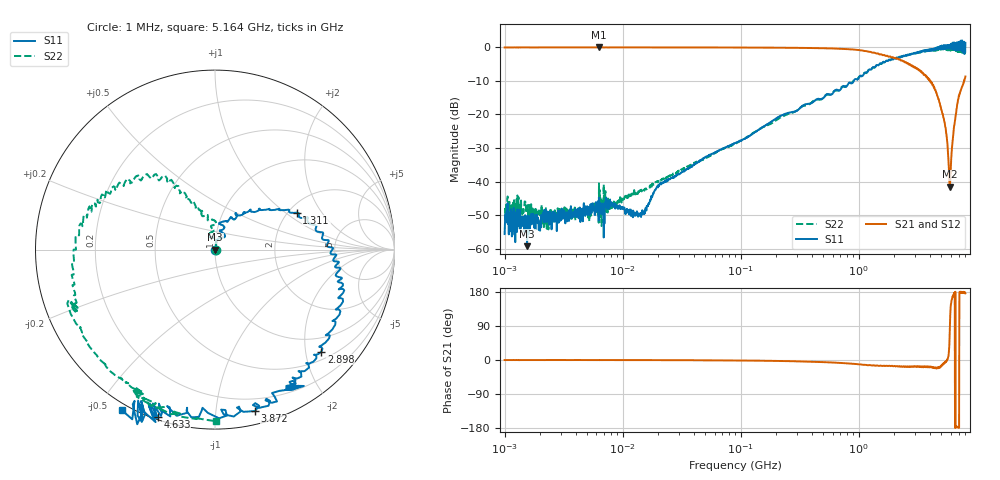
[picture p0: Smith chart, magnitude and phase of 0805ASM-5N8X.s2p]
!s-Parameter Generated by FASTRON Sdn. Bhd.
!FASTRON P/N : 0805ASM-5N8X
!Keysight Technologies: E5071C_MY46733604_B.14.02
!Date: Fri Jun 19 14:46:36 2026
!Version  :Rev00  Fri Jun 19 14:46:36 2026
!Data & Calibration Information:
!Freq  S11:SOLT2(ON)  S21:SOLT2(ON)  S12:SOLT2(ON)  S22:SOLT2(ON)
!PortZ  Port1:50+j0  Port2:50+j0
!When reading reference impedance value at option line is always used.
! Remarks : This data is being provided solely for informational purposes.
# Hz S dB R 50
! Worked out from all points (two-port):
!   1601 points, 1 MHz to 8 GHz, reference 50 ohm
!   highest |S21| = 0.01 dB at 6.301 MHz (marker M1); lowest = -41.5 dB at 5.918 GHz (marker M2)
!   |S21| within 3 dB of the highest: start of sweep to 1.886 GHz; 1.906 GHz to 1.955 GHz (49.23 MHz wide, 2.55 % of centre)
!   lowest |S11| = -59.2 dB at 1.55 MHz (marker M3), VSWR 1.00, Z = 50.1 - j0.0232 ohm
!   |S11| at or under -10 dB: start of sweep to 906.8 MHz
!   |S22| runs from -54.2 to -0.3 dB; largest |S21 - S12| = 0.0097
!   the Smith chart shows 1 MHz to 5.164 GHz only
!   S11 on the Smith chart (normalised r, x): 1 MHz: 1.00, -0.00; 1.311 GHz: 2.22, +1.22; 2.898 GHz: 0.67, -2.33; 3.872 GHz: 0.10, -1.27; 4.633 GHz: 0.01, -0.71; 5.164 GHz: -0.02, -0.58
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1000000  -55.60 -33.4  -0.04 -0.1  -0.03 -0.1  -49.20 -2.8
1066008  -52.60 13.6  -0.04 -0.1  -0.04 -0.0  -44.60 11.4
1550103  -59.20 -12.2  -0.03 -0.1  -0.03 -0.1  -48.00 -22.0
2173433  -48.90 24.8  -0.03 -0.1  -0.03 -0.0  -50.60 34.3
4479405  -49.80 21.3  -0.04 -0.1  -0.04 -0.1  -49.80 31.3
6301378  -44.80 33.3  0.01 -0.4  -0.00 -0.1  -40.50 41.1
1.414737e7  -49.30 64.4  -0.03 -0.3  -0.05 -0.3  -42.70 47.6
2.00676e7  -41.20 61.6  -0.04 -0.3  -0.05 -0.3  -39.90 66.8
8.994653e7  -28.50 78.6  -0.06 -1.3  -0.07 -1.2  -28.70 80.8
4.006501e8  -16.50 80.8  -0.22 -4.6  -0.22 -4.6  -16.30 87.9
1.310879e9  -6.02 24.3  -1.59 -14.2  -1.59 -14.3  -6.03 125.0
1.7949e9  -3.76 1.1  -2.81 -15.4  -2.81 -15.7  -3.73 145.0
2.472225e9  -2.49 -21.1  -4.53 -17.4  -4.59 -17.5  -2.46 165.0
2.89772e9  -1.71 -43.8  -5.61 -16.8  -5.69 -16.7  -1.96 -172.0
3.872345e9  -0.66 -76.1  -9.11 -17.4  -9.11 -17.6  -1.07 -142.0
4.632554e9  -0.14 -109.0  -14.50 -19.5  -14.50 -20.2  -0.84 -120.0
5.164399e9  0.30 -120.0  -20.10 -12.1  -20.10 -12.3  -0.39 -89.8
5.472309e9  -0.19 -137.0  -24.90 -5.7  -24.90 -5.9  -0.52 -65.5
5.752228e9  0.39 -142.0  -33.40 10.7  -33.50 10.6  -0.55 -56.9
5.918038e9  0.76 -142.0  -41.50 96.6  -41.50 96.3  -0.73 -60.3
6.72769e9  1.44 -150.0  -18.40 -175.0  -18.50 -176.0  -0.52 -5.1
8e9  1.32 156.0  -8.71 176.0  -8.62 176.0  -1.47 37.1
